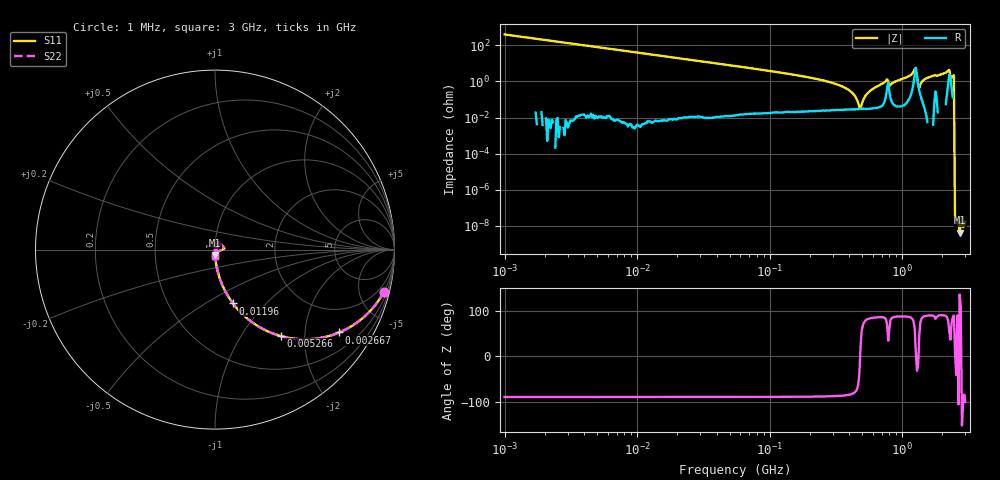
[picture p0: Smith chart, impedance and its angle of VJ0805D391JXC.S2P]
! VJ0805D391JXC
! DATE
! CORRECTED  DATA
# Hz  S  MA  R  50
!Freq	S11M	S11A	S21M	S21A	S12M	S12A	S22M	S22A
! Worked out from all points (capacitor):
!   401 points, 1 MHz to 3 GHz, reference 50 ohm
!   read as one part in series: C = 398 pF near 1.041 MHz
!   lowest |Z| = 4.18 nohm at 2.714 GHz (marker M1)
!   series resonance near 482.1 MHz, so ESL is about 270 pH
!   S11 on the Smith chart (normalised r, x): 1 MHz: 1.00, -7.99; 2.667 MHz: 1.00, -3.00; 5.266 MHz: 1.00, -1.52; 11.96 MHz: 1.00, -0.67; 3 GHz: 1.00, -0.07
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1000000  0.9701 -14.1  0.2428 76.0  0.2428 76.0  0.9701 -14.1
2666535  0.8318 -33.7  0.555 56.3  0.555 56.3  0.8318 -33.7
3823119  0.7225 -43.7  0.6912 46.3  0.6912 46.3  0.7225 -43.7
5266264  0.6044 -52.8  0.7966 37.2  0.7966 37.2  0.6044 -52.8
1.196486e7  0.3166 -71.5  0.9485 18.5  0.9485 18.5  0.3166 -71.5
1.461624e7  0.2635 -74.7  0.9646 15.3  0.9646 15.3  0.2635 -74.7
5.587962e7  0.07032 -85.9  0.9974 4.0  0.9974 4.0  0.07032 -85.9
2.094008e8  0.01548 -88.3  0.9997 0.9  0.9997 0.9  0.01548 -88.3
3.741707e8  0.004287 -86.1  0.9997 0.2  0.9997 0.2  0.004287 -86.1
4.219165e8  0.002261 -82.6  0.9997 0.1  0.9997 0.1  0.002261 -82.6
4.853736e8  0.0003287 20.4  0.9997 -0.0  0.9997 -0.0  0.0003287 20.4
5.81181e8  0.003277 84.2  0.9997 -0.2  0.9997 -0.2  0.003277 84.2
7.539071e8  0.01069 81.3  0.9984 -0.6  0.9984 -0.6  0.01069 81.3
8.005644e8  0.005491 60.6  0.9973 -0.3  0.9973 -0.3  0.005491 60.6
1.10276e9  0.01829 86.4  0.999 -1.0  0.999 -1.0  0.01829 86.4
1.218836e9  0.03436 75.2  0.9918 -1.9  0.9918 -1.9  0.03436 75.2
1.374365e9  0.007013 75.6  0.9983 -0.4  0.9983 -0.4  0.007013 75.6
1.54974e9  0.01581 88.9  0.9998 -0.9  0.9998 -0.9  0.01581 88.9
2.177892e9  0.03436 84.6  0.9973 -2.0  0.9973 -2.0  0.03436 84.6
2.407135e9  0.0195 84.9  0.9985 -1.1  0.9985 -1.1  0.0195 84.9
2.714296e9  0.02949 -88.5  1.001 -1.7  1.001 -1.7  0.02949 -88.5
3e9  0.0338 -87.4  1.002 -1.9  1.002 -1.9  0.0338 -87.4
